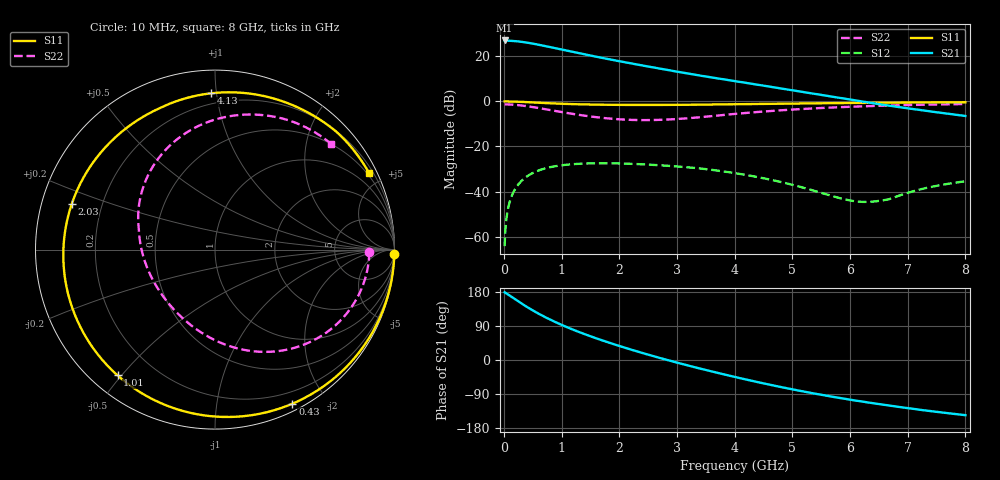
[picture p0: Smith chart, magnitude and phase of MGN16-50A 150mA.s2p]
! Port[1] = GATE
! Port[2] = DRAIN
! [Type]  S-parameter s2p file touchstone ver. 1.0
! [Object]  MGN16-50A
! [Bias]  150 mA
! [Version]  1.0
! [Date]  Thu May 28 11:03:16 2026
! [Source]  This file was created in JSC "ICC Milandr".
! [Disclaimer] Property of JSC "ICC Milandr". Unauthorized reproduction and/or distribution is strictly prohibited.
!  The file and the data are provided "AS IS" and with all faults and disclaim all warranties, express and implied, including
!  without limitation any implied warranties of merchantability, fitness for a particular purpose.
!  JSC "ICC Milandr" assumes no liability for:
!  1) the accuracy of the data provided;
!  2) the proper functioning of this data;
!  3) infringement of patents, copyrights or intellectual property rights resulting from the use of this data.
!  JSC "ICC Milandr" reserves the right to make changes to the products and the data without prior notice.
!  Please, be aware that your receipt and use of the file provided shall serve as acceptance of these terms and conditions.
!  If you do not accept these terms, you should return or destroy this file and any other accompanying information immediately.
# hz S ma R 12.5
! 2 Port Network Data from SP1.SP block
! freq  magS11  angS11  magS21  angS21  magS12  angS12  magS22  angS22
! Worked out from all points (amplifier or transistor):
!   800 points, 10 MHz to 8 GHz, reference 12.5 ohm
!   highest |S21| = 27.1 dB at 10 MHz (marker M1)
!   |S21| within 3 dB of that: start of sweep to 810.2 MHz
!   unconditionally stable (mu >= 1): 4.226 GHz to end of sweep
!   at 1.34 GHz: K = 0.19, MSG = 24.4 dB, |S12| = -27.6 dB
!   at 4.01 GHz: K = 0.89, MSG = 20.4 dB, |S12| = -31.9 dB
!   at 8 GHz: K = 1.09, MAG = 12.7 dB, |S12| = -35.4 dB
!   S11 on the Smith chart (normalised r, x): 10 MHz: 2, -75; 430 MHz: 0.07, -1.62; 1.01 GHz: 0.07, -0.49; 2.03 GHz: 0.09, +0.15; 4.13 GHz: 0.13, +0.97; 8 GHz: 0.40, +4.22
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1e7  0.9992 -1.5  22.57 178.8  0.0006127 82.1  0.8599 -0.9
4e7  0.9989 -6.2  22.49 175.7  0.002423 84.2  0.8593 -3.6
1e8  0.9967 -15.5  22.33 169.5  0.006011 79.2  0.8546 -9.0
1.9e8  0.9902 -29.2  21.89 160.2  0.0112 70.6  0.8407 -16.9
3.1e8  0.9771 -46.8  21.01 148.3  0.01755 59.4  0.8115 -27.1
4.3e8  0.9608 -63.3  19.9 137.0  0.02308 48.7  0.774 -36.6
5.5e8  0.9434 -78.8  18.67 126.4  0.02771 38.7  0.7321 -45.5
6.8e8  0.9251 -94.2  17.31 115.8  0.03178 28.6  0.6856 -54.5
8.5e8  0.9035 -112.4  15.59 103.0  0.03578 16.6  0.6273 -65.2
1.01e9  0.8865 -127.8  14.09 91.9  0.03845 6.3  0.5776 -74.6
1.17e9  0.8728 -141.6  12.75 81.7  0.04028 -3.3  0.5339 -83.5
1.35e9  0.8606 -155.7  11.41 71.0  0.04158 -13.3  0.4923 -93.0
1.66e9  0.8465 -176.6  9.48 54.0  0.04242 -29.0  0.4379 -109.1
2.03e9  0.8377 162.4  7.68 35.5  0.04187 -46.1  0.399 -128.3
2.35e9  0.835 147.1  6.449 20.7  0.04049 -59.8  0.3856 -145.1
2.68e9  0.8359 133.6  5.414 6.3  0.03845 -73.2  0.3891 -162.4
3.27e9  0.8446 113.5  3.989 -17.6  0.03377 -95.8  0.4311 168.5
4.01e9  0.8673 94.3  2.821 -45.0  0.02556 -114.6  0.5298 139.1
4.13e9  0.871 91.5  2.666 -49.2  0.02413 -117.1  0.5466 134.7
5.34e9  0.9067 66.4  1.495 -87.4  0.01075 -129.0  0.6985 96.7
6.67e9  0.9421 44.5  0.8061 -119.9  0.00672 -71.3  0.8118 65.6
8e9  0.9589 26.5  0.4755 -145.6  0.01689 -61.4  0.8754 42.3
